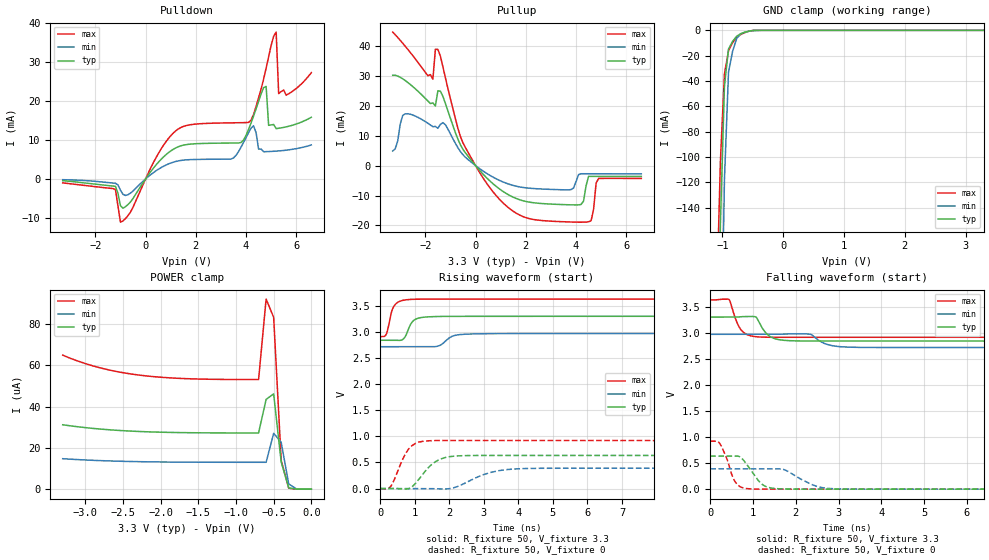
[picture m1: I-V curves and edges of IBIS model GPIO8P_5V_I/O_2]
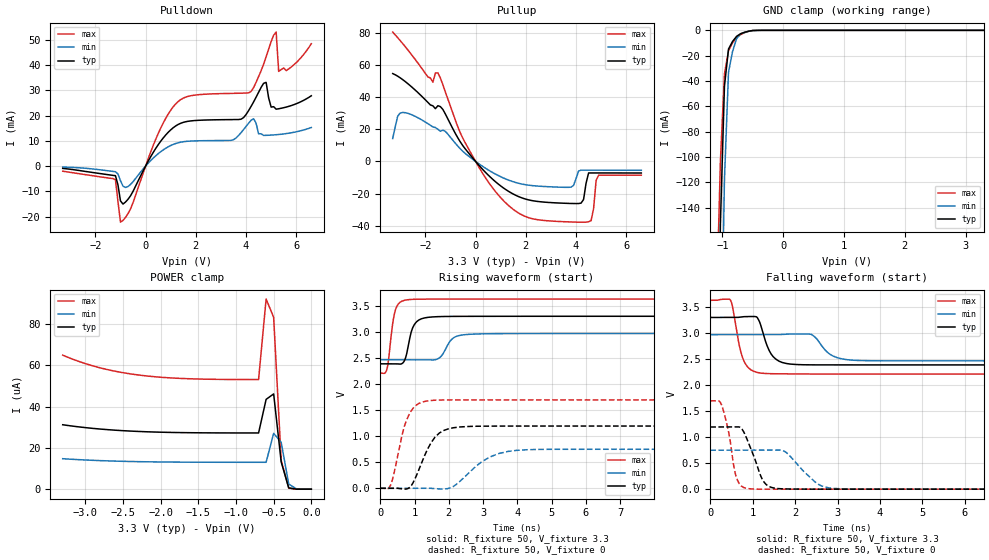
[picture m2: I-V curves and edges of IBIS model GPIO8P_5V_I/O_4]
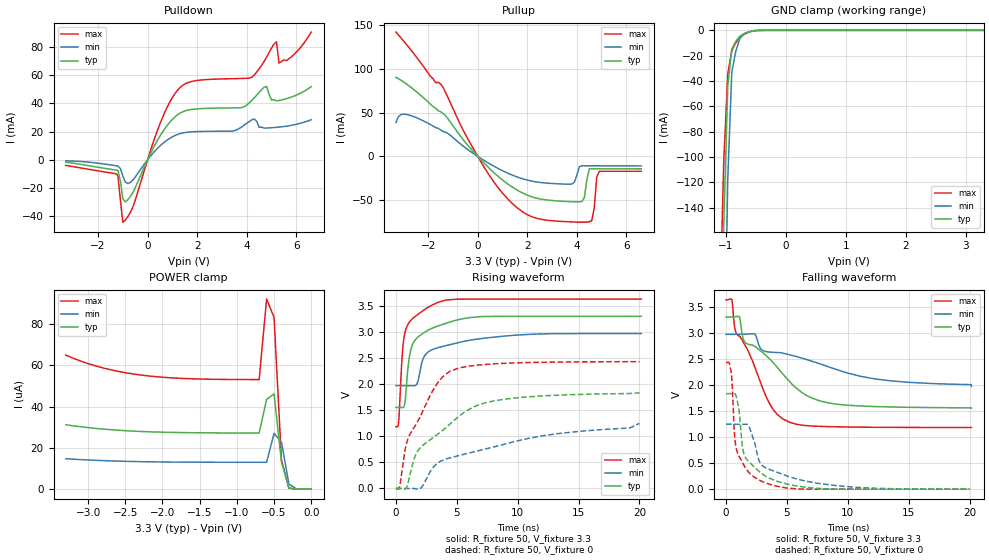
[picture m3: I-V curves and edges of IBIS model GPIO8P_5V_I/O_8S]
[IBIS ver]   4.2
[File name]   tm4c1236e6pm_64qfp_v0p0.ibs
[File Rev]   v0p0
[Date]   Oct 16, 2013
[Source]   simulation
[Notes]   IBIS models for 64qfp package with updated GPIO models
[Disclaimer] Please be aware that in the absence of a written agreement,
   Texas Instruments (TI) assumes no liability for: 1) the
   accuracy of the IBIS models provided to your company, 2) the
   proper functioning of these IBIS models in your design or for
   any resulting applications, or; 3) infringement of patents,
   copyrights, or intellectual property rights resulting from
   your use of these IBIS models. TI provides IBIS models as a
   service to our customers and therefore reserves the right to
   limit distribution of the IBIS models.
   This preliminary model does not contain all of the possible pad
   models for each of the pad types.  The most commonly used modes
   have been provided and the next update will include all of the
   pad model combinations.
   The only missing model that needs to be highlighted is the
   model for the USB D+ and D- GPIOs.  Currently only the USB
   functionality is provided on the D+ and D- pins.  Customers
   needing to model the PGIOs associated with these pins should
   check for a newer model.
[Copyright]   Property of Texas Instruments Incorporated. Unauthorized
   reproduction and/or distribution is strictly prohibited. This
   product is protected under copyright law and trade secret law
   as an unpublished work. Copyright (C) 2013, Texas Instruments
   Incorporated, all rights reserved. These commodities are under
   the U.S. Government distribution license control. As such,
   they are not to be re-exported without the prior approval of
   the U.S. Department of Commerce.
|   Component TM4C1236E6PM
[Component]   TM4C1236E6PM
[Manufacturer]   Texas Instruments Inc.
[Package]
| 64-pin QFP
| variable   typ   min   max
R_Pkg   1.54E-01   1.33E-01   1.88E-01
L_pkg   3.19E-09   2.78E-09   4.23E-09
C_pkg   8.38E-13   2.80E-13   9.90E-13
[Pin]   signal_name   model_name   R_pin   L_pin   C_pin
1   PB6   GPIO8P_5V   1.84E-01   3.33E-09   8.81E-13
2   VDDA   POWER
3   GNDA   GND
4   PB7   GPIO8P_5V   1.57E-01   2.94E-09   9.26E-13
5   PF4   GPIO8P_5V   1.48E-01   3.07E-09   8.85E-13
6   PE3   GPIO8P_5V   1.42E-01   2.92E-09   8.57E-13
7   PE2   GPIO8P_5V   1.37E-01   2.87E-09   8.36E-13
8   PE1   GPIO8P_5V   1.38E-01   2.89E-09   8.07E-13
9   PE0   GPIO8P_5V   1.39E-01   2.90E-09   7.97E-13
10   PD7   GPIO8P_5V   1.37E-01   2.83E-09   8.04E-13
11   VDD   POWER
12   GND   GND
13   PC7   GPIO8P_5V   1.33E-01   2.88E-09   8.79E-13
14   PC6   GPIO8P_5V   1.37E-01   2.97E-09   9.16E-13
15   PC5   GPIO8P_5V   1.43E-01   3.11E-09   9.48E-13
16   PC4   GPIO8P_5V   1.54E-01   3.26E-09   8.55E-13
17   PA0_U0Rx   GPIO8P_5V   1.58E-01   3.32E-09   8.54E-13
18   PA1_U0Tx   GPIO8P_5V   1.51E-01   3.11E-09   9.54E-13
19   PA2_SSI0Clk   GPIO8P_5V   1.48E-01   3.04E-09   9.29E-13
20   PA3_SSI0Fss   GPIO8P_5V   1.48E-01   3.04E-09   9.03E-13
21   PA4_SSI0Rx   GPIO8P_5V   1.50E-01   3.00E-09   8.84E-13
22   PA5_SSI0Tx   GPIO8P_5V   1.56E-01   2.97E-09   8.63E-13
23   PA6   GPIO8P_5V   1.60E-01   3.10E-09   8.54E-13
24   PA7   GPIO8P_5V   1.68E-01   2.98E-09   8.30E-13
25   VDDC   POWER
26   VDD   POWER
27   GND   GND
28   PF0   GPIO8P_5V   1.49E-01   3.03E-09   8.68E-13
29   PF1   GPIO8P_5V   1.50E-01   3.10E-09   9.06E-13
30   PF2   GPIO8P_5V   1.55E-01   3.21E-09   9.37E-13
31   PF3   GPIO8P_5V   1.62E-01   3.35E-09   9.55E-13
32   PG5   GPIO8P_5V   1.61E-01   3.37E-09   8.38E-13
33   PG4   GPIO8P_5V   1.88E-01   3.78E-09   8.89E-13
34   PG3   GPIO8P_5V   1.72E-01   3.53E-09   9.90E-13
35   PG2   GPIO8P_5V   1.59E-01   3.25E-09   9.49E-13
36   PG1   GPIO8P_5V   1.49E-01   3.10E-09   9.09E-13
37   PG0   GPIO8P_5V   1.42E-01   3.04E-09   8.61E-13
38   RST_n   RST_INPUT   1.55E-01   3.07E-09   8.54E-13
39   GND   GND
40   OSC0   NC
41   OSC1   NC
42   VDD   POWER
43   PD4   USB_PHY_DM   1.36E-01   2.87E-09   8.42E-13
44   PD5   USB_PHY_DP   1.38E-01   2.92E-09   8.62E-13
45   PB0_USB0ID   GPIO8P_5V   1.44E-01   3.06E-09   9.02E-13
46   PB1_USB0VBUS   GPIO8P_5V   1.53E-01   3.26E-09   9.40E-13
47   PB2_I2C0SCL   GPIO8P_5V   1.65E-01   3.51E-09   9.78E-13
48   PB3_I2C0SDA   GPIO8P_5V   1.80E-01   3.67E-09   8.78E-13
49   PC3_TDO_SWO   GPIO8P_5V   1.81E-01   3.74E-09   8.74E-13
50   PC2_TDI   GPIO8P_5V   1.68E-01   3.53E-09   9.76E-13
51   PC1_TMS_SWDIO  GPIO8P_5V   1.60E-01   3.29E-09   9.42E-13
52   PC0_TCK_SWCLK  GPIO8P_5V   1.54E-01   3.13E-09   8.95E-13
53   PD6   GPIO8P_5V   1.61E-01   3.01E-09   8.62E-13
54   VDD   POWER
55   GND   GND
56   VDDC   POWER
57   PB5   GPIO8P_5V   1.65E-01   2.96E-09   8.27E-13
58   PB4   GPIO8P_5V   1.58E-01   3.11E-09   8.46E-13
59   PE4   GPIO8P_5V   1.58E-01   3.15E-09   8.60E-13
60   PE5   GPIO8P_5V   1.52E-01   3.08E-09   8.84E-13
61   PD0   GPIO8P_5V   1.50E-01   3.07E-09   9.04E-13
62   PD1   GPIO8P_5V   1.50E-01   3.10E-09   9.29E-13
63   PD2   GPIO8P_5V   1.53E-01   3.24E-09   9.55E-13
64   PD3   GPIO8P_5V   1.60E-01   3.37E-09   8.43E-13
[Model Selector] GPIO8P_5V
GPIO8P_5V_I/O_2   2mA Output Buffer
GPIO8P_5V_I/O_4   4mA Output Buffer
GPIO8P_5V_I/O_8S   8mA Output Buffer with Slew Rate Control
GPIO8P_5V_I/O_8   8mA Output Buffer
GPIO8P_5V_I_WPU_2   2mA Input with Pull-Up
GPIO8P_5V_I_WPD_2   2mA Input with Pull-Down
GPIO8P_5V_I/O_OD_2   2mA Output Buffer with Open Drain
GPIO8P_5V_I/O_OD_4   4mA Output Buffer with Open Drain
GPIO8P_5V_I/O_OD_8S   8mA Output Buffer with Open Drain and Slew Rate Control
GPIO8P_5V_I/O_OD_8   8mA Output Buffer with Open Drain
[Model Selector] RST_INPUT
RST_IN   Input Model for the RST_n Pin
[Model Selector] USB_PHY_DP
fsdp_tx   Full Speed transmitter--12Mbps
lsdp_50pf_tx   Low speed transmitter--1.5Mbps driving 50pF cap load
lsdp_200pf_tx   Low speed transmitter--1.5Mbps driving 200pF cap load
lsdp_400pf_tx   Low speed transmitter--1.5Mbps driving 400pF cap load
lsdp_600pf_tx   Low speed transmitter--1.5Mbps driving 600pF cap load
fsdp_rx   Recieve mode--Open circuit during fs/ls recieve mode
[Model Selector] USB_PHY_DM
fsdm_tx   Full Speed transmitter--12Mbps
lsdm_50pf_tx   Low speed transmitter--1.5Mbps driving 50pF cap load
lsdm_200pf_tx   Low speed transmitter--1.5Mbps driving 200pF cap load
lsdm_400pf_tx   Low speed transmitter--1.5Mbps driving 400pF cap load
lsdm_600pf_tx 	 Low speed transmitter--1.5Mbps driving 600pF cap load
fsdm_rx   Recieve mode--Open circuit during fs/ls recieve mode
| Models and submodels in the file (23): GPIO8P_5V_I/O_2 (I/O), GPIO8P_5V_I/O_4 (I/O), GPIO8P_5V_I/O_8S (I/O), GPIO8P_5V_I/O_8 (I/O), GPIO8P_5V_I_WPU_2 (Input), GPIO8P_5V_I_WPD_2 (Input), GPIO8P_5V_I/O_OD_2 (I/O_open_drain), GPIO8P_5V_I/O_OD_4 (I/O_open_drain), GPIO8P_5V_I/O_OD_8S (I/O_open_drain), GPIO8P_5V_I/O_OD_8 (I/O_open_drain), RST_IN (Input), fsdp_tx (3-state), lsdp_50pf_tx (3-state), lsdp_200pf_tx (3-state), lsdp_400pf_tx (3-state), lsdp_600pf_tx (3-state), fsdp_rx (Input), fsdm_tx (3-state), lsdm_50pf_tx (3-state), lsdm_200pf_tx (3-state), lsdm_400pf_tx (3-state), lsdm_600pf_tx (3-state), fsdm_rx (Input)
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|   Model Cell GPIO8P_5V_I/O_2
[Model]   GPIO8P_5V_I/O_2
Model_type   I/O
Polarity   Non-Inverting
Enable   Active-Low
Vinl =  0.8
Vinh =  2
Cref =  15.0000pF
Rref =  100.0000M
Vref =  0V
Vmeas =  1.65
C_comp   4.711578p   4.034737p   5.423069p
[Model Spec]
Vinl   0.8   0.8   0.8
Vinh   2   2   2
[Temperature Range]   25   125   -40
[Voltage Range]   3.3   2.97   3.63
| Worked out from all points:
|   slope of the pulldown table from 0 to 0.495 V, typ, clamps not added: 118 ohm
|   slope of the pullup table from 0 to 0.495 V, typ, clamps not added: 109 ohm
|   GND clamp passes 1 mA (typ) near -0.59 V on its own axis
|   rising waveform, R_fixture 50, V_fixture 3.3: 20-80 % time 209ps typ, 304ps min, 170ps max; typ from 2.84 V to 3.3 V
|   rising waveform, R_fixture 50, V_fixture 0: 20-80 % time 527ps typ, 844ps min, 384ps max; typ from 0 V to 0.634 V
|   falling waveform, R_fixture 50, V_fixture 3.3: 20-80 % time 252ps typ, 337ps min, 213ps max; typ from 3.3 V to 2.84 V
|   falling waveform, R_fixture 50, V_fixture 0: 20-80 % time 342ps typ, 530ps min, 243ps max; typ from 0.634 V to 0 V
| Nom Voltages:
|   VDDC=1.2, VDD=3.3, GND=0
| Min Voltages:
|   VDDC=1.08, VDD=2.97, GND=0
| Max Voltages:
|   VDDC=1.32, VDD=3.63, GND=0
[POWER_clamp]
|   voltage   I(typ)   I(min)   I(max)
-3.3V     31.22uA    14.76uA    64.95uA
-3.1V     30.25uA    14.33uA    62.09uA
-2.8V     29.13uA    13.84uA    58.77uA
-2.3V     27.98uA    13.34uA    55.36uA
-1.7V     27.4uA     13.1uA     53.62uA
-700mV    27.24uA    13.03uA    53.12uA
-600mV    43.52uA    13.03uA    92.14uA
-500mV    46.16uA    27.05uA    83.3uA
-400mV    13.21uA    22.74uA    13.98uA
-300mV    630.7nA    2.501uA    480.9nA
-200mV    23.21nA    190.8nA    10.65nA
0V        660.4pA    10.19nA    564.9pA
[Pulldown]
|   voltage   I(typ)   I(min)   I(max)
-3.3V     -450.7uA   -192.2uA   -1.006mA
-1.2V     -1.893mA   -1.109mA   -2.697mA
-1V       -6.866mA   -2.892mA   -11.1mA
1.2V      7.958mA    4.478mA    12.33mA
3.5V      9.211mA    5.381mA    14.4mA
4.2V      14.36mA    13.04mA    15.06mA
4.5V      19.92mA    7.668mA    20.83mA
4.8V      23.73mA    7.004mA    28.42mA
4.9V      13.75mA    7.03mA     31.35mA
5.2V      12.91mA    7.14mA     37.68mA
5.3V      13mA       7.19mA     21.9mA
6.6V      15.82mA    8.714mA    27.27mA
[Pullup]
|   voltage   I(typ)   I(min)   I(max)
-3.3V     30.16mA    4.863mA    44.59mA
-2.9V     28.98mA    16.78mA    40.86mA
-1.7V     20.92mA    12.98mA    28.86mA
-1.6V     19.91mA    13.09mA    38.88mA
-1.5V     24.98mA    12.47mA    38.79mA
-500mV    5.386mA    3.597mA    7.551mA
1.6V      -10.92mA   -6.844mA   -15.8mA
3.8V      -13.1mA    -8.018mA   -18.83mA
4.2V      -12.99mA   -2.721mA   -18.9mA
4.5V      -3.591mA   -2.724mA   -18.76mA
4.9V      -3.59mA    -2.729mA   -4.279mA
6.6V      -3.606mA   -2.757mA   -4.278mA
[GND_clamp]
|   voltage   I(typ)   I(min)   I(max)
-3.3V     -16.3A     -15.26A    -17.13A
-1.1V     -340.4mA   -570.5mA   -222.8mA
-1.033V   -152.7mA   -296.8mA   -103.3mA
-966.7mV  -44.18mA   -117.7mA   -34.4mA
-900mV    -14.77mA   -33.12mA   -16.14mA
-833.3mV  -8.752mA   -16.68mA   -9.833mA
-766.7mV  -4.716mA   -6.551mA   -5.563mA
-700mV    -2.657mA   -2.741mA   -3.333mA
-566.7mV  -672.8uA   -727.2uA   -724.4uA
-433.3mV  -51.87uA   -90.8uA    -37.79uA
3.3V      660.4pA    5.308uA    422.7pA
[Ramp]
| variable   typ   min   max
dV/dt_f 0.28269897/0.25386606n 0.15654957/0.33829046n 0.43992818/0.21519855n
dV/dt_r 0.38699946/0.53401128n 0.23880101/0.85366195n 0.55927105/0.38819382n
R_load = 50
[Rising Waveform]
R_fixture = 50
V_fixture = 3.3
V_fixture_min = 2.97
V_fixture_max = 3.63
|   time   V(typ)   V(min)   V(max)
0s        2.841V     2.717V     2.912V
178.1ps   2.841V     2.717V     2.965V
341.5ps   2.841V     2.717V     3.419V
428.4ps   2.841V     2.717V     3.523V
687.2ps   2.877V     2.717V     3.61V
833.7ps   3.083V     2.717V     3.622V
1.166ns   3.274V     2.717V     3.628V
2.143ns   3.299V     2.931V     3.63V
2.818ns   3.299V     2.964V     3.63V
20.12ns   3.3V       2.97V      3.63V
[Rising Waveform]
R_fixture = 50
V_fixture = 0
V_fixture_min = 0
V_fixture_max = 0
|   time   V(typ)   V(min)   V(max)
0s        0V         0V         0V
320.1ps   0V         0V         57.85mV
634.7ps   -8.112mV   0V         543.5mV
833.3ps   0V         0V         764.8mV
1.337ns   360.6mV    0V         913.4mV
1.604ns   518.1mV    -4.493mV   919.6mV
2.025ns   613mV      0V         920.5mV
3.179ns   634.6mV    306.6mV    919.8mV
4.221ns   634.3mV    384.5mV    919.7mV
20.01ns   634.3mV    389.8mV    919.8mV
[Falling Waveform]
R_fixture = 50
V_fixture = 3.3
V_fixture_min = 2.97
V_fixture_max = 3.63
|   time   V(typ)   V(min)   V(max)
0s        3.3V       2.97V      3.63V
436.2ps   3.3V       2.97V      3.639V
720.2ps   3.308V     2.97V      3.054V
1.059ns   3.305V     2.97V      2.925V
1.179ns   3.141V     2.97V      2.917V
1.464ns   2.899V     2.97V      2.913V
2.039ns   2.843V     2.978V     2.913V
2.834ns   2.842V     2.755V     2.913V
3.318ns   2.841V     2.722V     2.913V
20.12ns   2.841V     2.717V     2.913V
[Falling Waveform]
R_fixture = 50
V_fixture = 0
V_fixture_min = 0
V_fixture_max = 0
|   time   V(typ)   V(min)   V(max)
0s        634.3mV    389.8mV    919.8mV
229.2ps   634.3mV    389.8mV    866.6mV
521.5ps   634.1mV    389.8mV    237.1mV
636.8ps   634.8mV    389.8mV    84.64mV
1.041ns   261.6mV    389.8mV    0V
1.409ns   23.56mV    389.7mV    0V
1.746ns   3.625mV    368.6mV    0V
2.48ns    0V         56.31mV    0V
3.006ns   0V         5.108mV    0V
20.01ns   0V         0V         0V
|   Model Cell GPIO8P_5V_I/O_4
[Model]   GPIO8P_5V_I/O_4
Model_type   I/O
Polarity   Non-Inverting
Enable   Active-Low
Vinl =  0.8
Vinh =  2
Cref =  15.0000pF
Rref =  100.0000M
Vref =  0V
Vmeas =  1.65
C_comp   4.711578p   4.034737p   5.423069p
[Model Spec]
Vinl   0.8   0.8   0.8
Vinh   2   2   2
[Temperature Range]   25   125   -40
[Voltage Range]   3.3   2.97   3.63
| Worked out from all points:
|   slope of the pulldown table from 0 to 0.495 V, typ, clamps not added: 59.3 ohm
|   slope of the pullup table from 0 to 0.495 V, typ, clamps not added: 59.2 ohm
|   GND clamp passes 1 mA (typ) near -0.59 V on its own axis
|   rising waveform, R_fixture 50, V_fixture 3.3: 20-80 % time 208ps typ, 290ps min, 166ps max; typ from 2.39 V to 3.3 V
|   rising waveform, R_fixture 50, V_fixture 0: 20-80 % time 516ps typ, 844ps min, 381ps max; typ from 0 V to 1.2 V
|   falling waveform, R_fixture 50, V_fixture 3.3: 20-80 % time 259ps typ, 347ps min, 216ps max; typ from 3.3 V to 2.39 V
|   falling waveform, R_fixture 50, V_fixture 0: 20-80 % time 329ps typ, 535ps min, 221ps max; typ from 1.2 V to 0 V
| Nom Voltages:
|   VDDC=1.2, VDD=3.3, GND=0
| Min Voltages:
|   VDDC=1.08, VDD=2.97, GND=0
| Max Voltages:
|   VDDC=1.32, VDD=3.63, GND=0
[POWER_clamp]
|   voltage   I(typ)   I(min)   I(max)
-3.3V     31.22uA    14.76uA    64.95uA
-3.1V     30.25uA    14.33uA    62.09uA
-2.8V     29.13uA    13.84uA    58.77uA
-2.3V     27.98uA    13.34uA    55.36uA
-1.7V     27.4uA     13.1uA     53.62uA
-700mV    27.24uA    13.03uA    53.12uA
-600mV    43.52uA    13.03uA    92.14uA
-500mV    46.16uA    27.05uA    83.3uA
-400mV    13.21uA    22.74uA    13.98uA
-300mV    630.7nA    2.501uA    480.9nA
-200mV    23.21nA    190.8nA    10.65nA
0V        660.4pA    10.19nA    564.9pA
[Pulldown]
|   voltage   I(typ)   I(min)   I(max)
-3.3V     -901.6uA   -384.4uA   -2.013mA
-1.2V     -3.786mA   -2.218mA   -5.418mA
-1V       -13.75mA   -5.79mA    -22.19mA
-700mV    -13.13mA   -8.08mA    -18.83mA
1.3V      16.5mA     9.253mA    25.59mA
3.5V      18.42mA    10.46mA    28.8mA
4.2V      23.61mA    18.14mA    29.55mA
4.8V      33.14mA    12.18mA    43.24mA
5V        23.36mA    12.28mA    49.33mA
5.2V      22.53mA    12.43mA    53.05mA
5.3V      22.7mA     12.52mA    37.48mA
6.6V      27.85mA    15.27mA    48.43mA
[Pullup]
|   voltage   I(typ)   I(min)   I(max)
-3.3V     54.59mA    14.22mA    80.39mA
-3.1V     52.96mA    28.24mA    76.9mA
-2.6V     47.05mA    29.37mA    67.36mA
-1.7V     34.57mA    21.42mA    49.25mA
-1.5V     34.64mA    19.97mA    55.03mA
100mV     -1.815mA   -1.128mA   -2.736mA
1.8V      -22.4mA    -13.91mA   -32.86mA
3.8V      -26.14mA   -15.97mA   -37.63mA
4.2V      -25.93mA   -5.421mA   -37.77mA
4.5V      -7.168mA   -5.427mA   -37.49mA
4.9V      -7.166mA   -5.439mA   -8.552mA
6.6V      -7.2mA     -5.497mA   -8.551mA
[GND_clamp]
|   voltage   I(typ)   I(min)   I(max)
-3.3V     -16.3A     -15.26A    -17.13A
-1.1V     -340.4mA   -570.5mA   -222.8mA
-1.033V   -152.7mA   -296.8mA   -103.3mA
-966.7mV  -44.18mA   -117.7mA   -34.4mA
-900mV    -14.77mA   -33.12mA   -16.14mA
-833.3mV  -8.752mA   -16.68mA   -9.833mA
-766.7mV  -4.716mA   -6.551mA   -5.563mA
-700mV    -2.657mA   -2.741mA   -3.333mA
-566.7mV  -672.8uA   -727.2uA   -724.4uA
-433.3mV  -51.87uA   -90.8uA    -37.79uA
3.3V      660.4pA    5.308uA    422.7pA
[Ramp]
| variable   typ   min   max
dV/dt_f  0.5587141/0.26045662n 0.31023858/0.352185n  0.86504244/0.21760119n
dV/dt_r 0.72667108/0.52198411n 0.45768162/0.8533017n   1.027789/0.38356156n
R_load = 50
[Rising Waveform]
R_fixture = 50
V_fixture = 3.3
V_fixture_min = 2.97
V_fixture_max = 3.63
|   time   V(typ)   V(min)   V(max)
0s        2.388V     2.466V     2.211V
198.6ps   2.388V     2.466V     2.297V
375ps     2.388V     2.466V     3.219V
457.4ps   2.387V     2.466V     3.451V
692.2ps   2.433V     2.466V     3.604V
849.4ps   2.842V     2.466V     3.621V
982.8ps   3.13V      2.466V     3.626V
1.222ns   3.257V     2.466V     3.629V
2.761ns   3.299V     2.959V     3.63V
20.01ns   3.3V       2.97V      3.63V
[Rising Waveform]
R_fixture = 50
V_fixture = 0
V_fixture_min = 0
V_fixture_max = 0
|   time   V(typ)   V(min)   V(max)
0s        0V         0V         0V
299.4ps   0V         0V         59.61mV
695.5ps   -16.31mV   0V         1.174V
860.4ps   17.92mV    0V         1.439V
1.44ns    827.9mV    0V         1.683V
1.727ns   1.062V     -12.61mV   1.693V
2.127ns   1.161V     33.95mV    1.695V
3.187ns   1.193V     597.4mV    1.696V
4.256ns   1.194V     739mV      1.696V
20.15ns   1.195V     748.9mV    1.696V
[Falling Waveform]
R_fixture = 50
V_fixture = 3.3
V_fixture_min = 2.97
V_fixture_max = 3.63
|   time   V(typ)   V(min)   V(max)
0s        3.3V       2.97V      3.63V
471.4ps   3.3V       2.97V      3.639V
817.4ps   3.316V     2.97V      2.422V
1.099ns   3.305V     2.97V      2.245V
1.273ns   2.918V     2.97V      2.224V
1.545ns   2.499V     2.97V      2.218V
2.126ns   2.392V     2.982V     2.214V
2.889ns   2.388V     2.56V      2.212V
3.475ns   2.388V     2.474V     2.212V
20.01ns   2.388V     2.466V     2.212V
[Falling Waveform]
R_fixture = 50
V_fixture = 0
V_fixture_min = 0
V_fixture_max = 0
|   time   V(typ)   V(min)   V(max)
0s        1.195V     748.8mV    1.697V
263ps     1.195V     748.8mV    1.625V
432ps     1.195V     748.8mV    1.1V
625.9ps   1.196V     748.8mV    202.3mV
899ps     892.7mV    748.8mV    9.985mV
1.272ns   130mV      748.8mV    0V
1.676ns   7.24mV     748.3mV    0V
2.497ns   0V         122.3mV    0V
3.021ns   0V         9.096mV    0V
20.15ns   0V         0V         0V
|   Model Cell GPIO8P_5V_I/O_8S
[Model]   GPIO8P_5V_I/O_8S
Model_type   I/O
Polarity   Non-Inverting
Enable   Active-Low
Vinl =  0.8
Vinh =  2
Cref =  15.0000pF
Rref =  100.0000M
Vref =  0V
Vmeas =  1.65
C_comp   4.711578p   4.034737p   5.423069p
[Model Spec]
Vinl   0.8   0.8   0.8
Vinh   2   2   2
[Temperature Range]   25   125   -40
[Voltage Range]   3.3   2.97   3.63
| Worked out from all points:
|   slope of the pulldown table from 0 to 0.495 V, typ, clamps not added: 29.7 ohm
|   slope of the pullup table from 0 to 0.495 V, typ, clamps not added: 34.2 ohm
|   GND clamp passes 1 mA (typ) near -0.59 V on its own axis
|   rising waveform, R_fixture 50, V_fixture 3.3: 20-80 % time 1.23ns typ, 2.77ns min, 657ps max; typ from 1.55 V to 3.3 V
|   rising waveform, R_fixture 50, V_fixture 0: 20-80 % time 4.41ns typ, 9.1ns min, 2.62ns max; typ from 0 V to 1.83 V
|   falling waveform, R_fixture 50, V_fixture 3.3: 20-80 % time 4.63ns typ, 8.26ns min, 2.82ns max; typ from 3.3 V to 1.55 V
|   falling waveform, R_fixture 50, V_fixture 0: 20-80 % time 1.5ns typ, 2.86ns min, 884ps max; typ from 1.83 V to 0 V
| Nom Voltages:
|   VDDC=1.2, VDD=3.3, GND=0
| Min Voltages:
|   VDDC=1.08, VDD=2.97, GND=0
| Max Voltages:
|   VDDC=1.32, VDD=3.63, GND=0
[POWER_clamp]
|   voltage   I(typ)   I(min)   I(max)
-3.3V     31.22uA    14.76uA    64.95uA
-3.1V     30.25uA    14.33uA    62.09uA
-2.8V     29.13uA    13.84uA    58.77uA
-2.3V     27.98uA    13.34uA    55.36uA
-1.7V     27.4uA     13.1uA     53.62uA
-700mV    27.24uA    13.03uA    53.12uA
-600mV    43.52uA    13.03uA    92.14uA
-500mV    46.16uA    27.05uA    83.3uA
-400mV    13.21uA    22.74uA    13.98uA
-300mV    630.7nA    2.501uA    480.9nA
-200mV    23.21nA    190.8nA    10.65nA
0V        660.3pA    10.19nA    564.9pA
[Pulldown]
|   voltage   I(typ)   I(min)   I(max)
-3.3V     -1.804mA   -768.9uA   -4.029mA
-1.2V     -7.576mA   -4.438mA   -10.94mA
-1V       -27.56mA   -11.61mA   -44.39mA
-700mV    -26.23mA   -16.15mA   -37.6mA
500mV     16.83mA    9.794mA    25.59mA
1.3V      32.99mA    18.5mA     51.14mA
3.5V      36.85mA    20.6mA     57.6mA
4.2V      42.1mA     28.33mA    58.55mA
4.8V      51.96mA    22.52mA    72.86mA
5.2V      41.77mA    23mA       83.78mA
5.3V      42.1mA     23.17mA    68.63mA
6.6V      51.87mA    28.39mA    90.67mA
[Pullup]
|   voltage   I(typ)   I(min)   I(max)
-3.3V     90.55mA    38.78mA    142.4mA
-2.4V     72.32mA    43.42mA    111.1mA
-1.4V     49.16mA    28.51mA    79.12mA
600mV     -17.27mA   -10.43mA   -27.2mA
2V        -44.4mA    -27.17mA   -66.73mA
3.8V      -51.96mA   -31.62mA   -75.08mA
4.2V      -51.61mA   -10.74mA   -75.41mA
4.5V      -14.27mA   -10.76mA   -74.89mA
4.6V      -14.27mA   -10.77mA   -73.6mA
4.8V      -14.27mA   -10.78mA   -23.97mA
4.9V      -14.27mA   -10.79mA   -17.08mA
6.6V      -14.35mA   -10.92mA   -17.08mA
[GND_clamp]
|   voltage   I(typ)   I(min)   I(max)
-3.3V     -16.3A     -15.26A    -17.13A
-1.1V     -340.4mA   -570.5mA   -222.8mA
-1.033V   -152.7mA   -296.8mA   -103.3mA
-966.7mV  -44.18mA   -117.7mA   -34.4mA
-900mV    -14.77mA   -33.12mA   -16.14mA
-833.3mV  -8.752mA   -16.68mA   -9.833mA
-766.7mV  -4.716mA   -6.551mA   -5.563mA
-700mV    -2.657mA   -2.741mA   -3.333mA
-566.7mV  -672.8uA   -727.2uA   -724.4uA
-433.3mV  -51.87uA   -90.8uA    -37.79uA
3.3V      660.3pA    5.308uA    422.7pA
[Ramp]
| variable   typ   min   max
dV/dt_f  1.0557963/4.6216941n 0.60488119/8.2398767n  1.4782959/2.8219071n
dV/dt_r  1.1075872/4.4039012n 0.75620404/9.0634394n  1.4663476/2.6218461n
R_load = 50
[Rising Waveform]
R_fixture = 50
V_fixture = 3.3
V_fixture_min = 2.97
V_fixture_max = 3.63
|   time   V(typ)   V(min)   V(max)
0s        1.553V     1.971V     1.182V
219.8ps   1.553V     1.971V     1.259V
549.8ps   1.55V      1.971V     2.656V
813.3ps   1.809V     1.971V     3.049V
1.018ns   2.375V     1.971V     3.158V
1.326ns   2.741V     1.971V     3.248V
1.727ns   2.884V     2.004V     3.323V
2.94ns    3.067V     2.656V     3.512V
7.005ns   3.294V     2.873V     3.63V
20.16ns   3.3V       2.97V      3.63V
[Rising Waveform]
R_fixture = 50
V_fixture = 0
V_fixture_min = 0
V_fixture_max = 0
|   time   V(typ)   V(min)   V(max)
0s        0V         0V         0V
296.6ps   0V         0V         32.98mV
750.1ps   -12.44mV   0V         741.7mV
1.068ns   177.6mV    0V         998.7mV
1.849ns   738.5mV    -11.92mV   1.308V
3.143ns   987.7mV    425.3mV    1.922V
4.391ns   1.226V     583.2mV    2.242V
6.234ns   1.544V     690.6mV    2.35V
8.039ns   1.678V     795.2mV    2.388V
20.01ns   1.831V     1.248V     2.43V
[Falling Waveform]
R_fixture = 50
V_fixture = 3.3
V_fixture_min = 2.97
V_fixture_max = 3.63
|   time   V(typ)   V(min)   V(max)
0s        3.3V       2.97V      3.63V
473.3ps   3.3V       2.97V      3.639V
717.3ps   3.307V     2.97V      3.089V
1.083ns   3.31V      2.97V      2.936V
1.501ns   2.834V     2.97V      2.79V
2.371ns   2.739V     2.975V     2.336V
3.475ns   2.522V     2.631V     1.686V
4.628ns   2.221V     2.611V     1.353V
8.542ns   1.649V     2.337V     1.199V
20.16ns   1.553V     1.971V     1.182V
[Falling Waveform]
R_fixture = 50
V_fixture = 0
V_fixture_min = 0
V_fixture_max = 0
|   time   V(typ)   V(min)   V(max)
0s        1.831V     1.246V     2.43V
252.7ps   1.831V     1.246V     2.424V
434.2ps   1.831V     1.246V     2.213V
698.6ps   1.833V     1.246V     1.039V
871.5ps   1.748V     1.246V     748.2mV
1.478ns   667.5mV    1.246V     454.5mV
1.94ns    508.6mV    1.171V     304.9mV
2.697ns   343.8mV    555.6mV    176.4mV
7.541ns   15.64mV    111.8mV    0V
20.01ns   0V         0V         0V
